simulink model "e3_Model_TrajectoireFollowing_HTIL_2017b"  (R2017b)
settings: Solver=FixedStepAuto  StartTime=0.0  StopTime=100  FixedStep=sampleTime  RelTol=1e-3  EnableMultiTasking=on
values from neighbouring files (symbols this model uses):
  k_d_x = 1.5    [StartSimulation.m]    (also in startSimulation.m; start.m = 1.65)
  k_d_y = 1.5    [StartSimulation.m]    (also in startSimulation.m; start.m = 1.52)
  k_d_yaw = 1    [StartSimulation.m]    (also in startSimulation.m; start.m)
  k_d_z = 0.5    [StartSimulation.m]    (also in startSimulation.m; start.m)
  k_i_x = 0.01    [StartSimulation.m]    (also in startSimulation.m; start.m = 0.9)
  k_i_y = 0.01    [StartSimulation.m]    (also in startSimulation.m; start.m = 0.91)
  k_i_yaw = 0.01    [StartSimulation.m]    (also in startSimulation.m; start.m)
  k_i_z = 0.01    [StartSimulation.m]    (also in startSimulation.m; start.m)
  k_p_x = 1.2    [StartSimulation.m]    (also in startSimulation.m; start.m = 1.9)
  k_p_y = 1.5    [StartSimulation.m]    (also in startSimulation.m; start.m = 1.9)
  k_p_yaw = 2    [StartSimulation.m]    (also in startSimulation.m; start.m)
  k_p_z = 2    [StartSimulation.m]    (also in startSimulation.m; start.m)
  saturation_psi = 2    [StartSimulation.m]    (also in startSimulation.m; start.m)
  saturation_x = 2    [StartSimulation.m]    (also in startSimulation.m; start.m)
  saturation_y = 2    [StartSimulation.m]    (also in startSimulation.m; start.m)
  saturation_z = 2    [StartSimulation.m]    (also in startSimulation.m; start.m)
libraries: simulink x37, aerolibanimutils x2, etargetslib x2

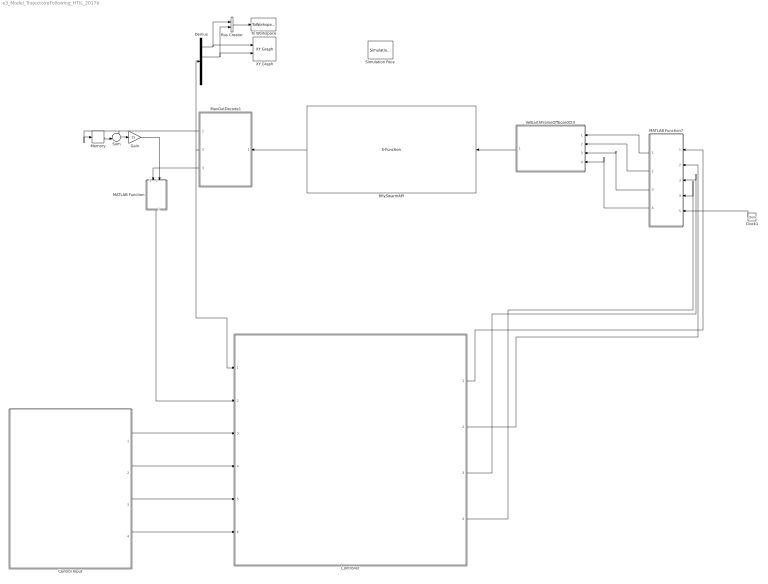
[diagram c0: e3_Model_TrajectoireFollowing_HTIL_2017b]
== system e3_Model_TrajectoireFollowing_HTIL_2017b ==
  Bus Creator : BusCreator  Inputs=2
  Clock1 : Clock
  Control Input : Subsystem
  Controller : Subsystem
  Demux : Demux
  Gain : Gain  Gain=25
  MATLAB Function : MATLAB Function  TreatAsAtomicUnit=on
  MATLAB Function7 : MATLAB Function  TreatAsAtomicUnit=on
  MavOutDecode1 : MATLAB Function  TreatAsAtomicUnit=on
  Memory : Memory
  RflySwarmAPI : S-Function  FunctionName=RflyUdpFast  Parameters=port,num,modeValue,T,ip  SFunctionDeploymentMode=off  EnableBusSupport=off  mask(UDP Receive){ip=255.255.255.255, port=20100, num=1, mode=FullData Mode, T=1/25, modeValue=0}
      mask prompts: ip "UDP IP Address"; port "UDP Port"; num "vehicle Number"; mode "UDP Mode"; T "Sample Time"
      mask help: This block receives bytes from an UDP/IP connection. The first parameter is the UDP port on the first CopterSim App The second parameter is the total vehicle number The third parameter is the data mode. check the help button for the definition
      mask init:
      | if strcmp(mode,'FullData Mode')
      |     modeValue = 0;
      | elseif strcmp(mode,'SimpleData Mode') 
      |     modeValue = 1;
      | elseif strcmp(mode,'UltraSimple Mode') 
      |     modeValue = 2;
      | else
      |     modeValue = 0;
      | end
  Simulation Pace : aerolibanimutils/Simulation Pace  SimulationPace=1  SleepMode=MATLAB Thread  OutputPaceError=off  SampleTime=-1
  Sum : Sum  Inputs=+-|
  To Workspace : ToWorkspace  VariableName=Pos  SaveFormat=Timeseries  SampleTime=-1
  VelEarthFrameOffboardCtrl : Subsystem
  XY Graph : simulink/Sinks/XY Graph  xmin=-1  xmax=1  ymin=-1  ymax=1  st=-1
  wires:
  Controller/1(Controller Output X) -> MATLAB Function7/1(X)
  Controller/2(Controller Output Y) -> MATLAB Function7/2(Y)
  Controller/3(Controller Output H) -> MATLAB Function7/3(H)
  Controller/4(Controller Output Psi) -> MATLAB Function7/4(Psi)
  Control Input/1(ux) -> Controller/3(Control input X)
  Control Input/2(uy) -> Controller/4(Control input Y)
  Control Input/3(uz) -> Controller/5(Control input H)
  Control Input/4(upsi) -> Controller/6(Control input Psi)
  RflySwarmAPI/1 -> MavOutDecode1/1(u)
  VelEarthFrameOffboardCtrl/1(Out1) -> RflySwarmAPI/1
  Clock1/1 -> MATLAB Function7/5(t)
  MATLAB Function7/4(p1) -> VelEarthFrameOffboardCtrl/4(yawRate_rads)
  MATLAB Function7/3(h1) -> VelEarthFrameOffboardCtrl/3(VeZ_ms)
  MATLAB Function7/2(y1) -> VelEarthFrameOffboardCtrl/2(VeY_ms)
  MATLAB Function7/1(x1) -> VelEarthFrameOffboardCtrl/1(VeX_ms)
  MavOutDecode1/2(localPos) -> Demux/1, Controller/1(Feedback Position)
  Demux/1 -> Bus Creator/1, XY Graph/1
  Demux/2 -> Bus Creator/2, XY Graph/2
  MavOutDecode1/1(Psi) -> Memory/1, Sum/1
  Memory/1 -> Sum/2
  Sum/1 -> Gain/1
  Gain/1 -> MATLAB Function/2(psi)
  MavOutDecode1/3(localVel) -> MATLAB Function/1(v)
  MATLAB Function/1(y) -> Controller/2(Feedback Velocity)
  Bus Creator/1 -> To Workspace/1

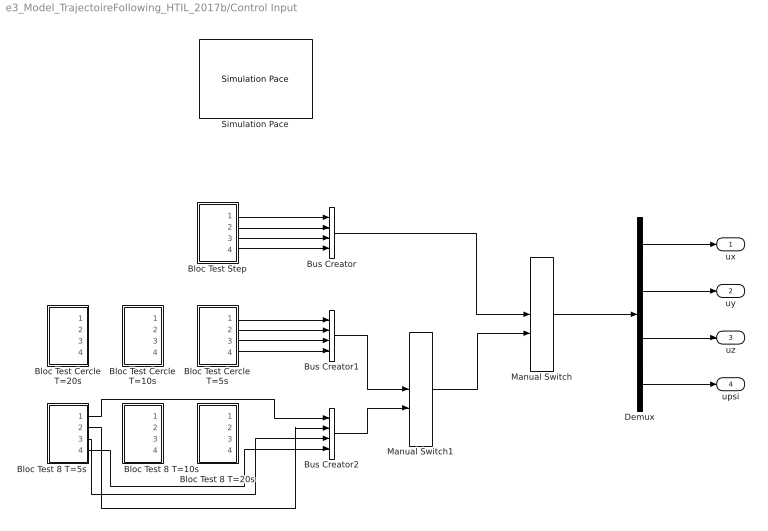
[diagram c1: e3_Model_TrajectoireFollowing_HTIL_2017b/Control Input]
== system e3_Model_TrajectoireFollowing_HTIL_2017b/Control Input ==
  Bloc Test 8 T=10s : Subsystem
  Bloc Test 8 T=20s : Subsystem
  Bloc Test 8 T=5s : Subsystem
  Bloc Test Cercle T=10s : Subsystem
  Bloc Test Cercle T=20s : Subsystem
  Bloc Test Cercle T=5s : Subsystem
  Bloc Test Step : Subsystem
  Bus Creator : BusCreator  Inputs=4
  Bus Creator1 : BusCreator  Inputs=4
  Bus Creator2 : BusCreator  Inputs=4
  Demux : Demux
  Manual Switch : ManualSwitch  CurrentSetting=0
  Manual Switch1 : ManualSwitch
  Simulation Pace : aerolibanimutils/Simulation Pace  Commented=on  SimulationPace=100  SleepMode=MATLAB Thread  OutputPaceError=off  SampleTime=-1
  ux : Outport
  uy : Outport  Port=2
  uz : Outport  Port=3
  upsi : Outport  Port=4
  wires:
  Demux/2 -> uy/1
  Demux/1 -> ux/1
  Bloc Test Step/2(uy) -> Bus Creator/2
  Demux/3 -> uz/1
  Demux/4 -> upsi/1
  Bloc Test Step/4(upsi) -> Bus Creator/4
  Bloc Test Step/3(uz) -> Bus Creator/3
  Bloc Test Step/1(ux) -> Bus Creator/1
  Bus Creator/1 -> Manual Switch/1
  Bus Creator1/1 -> Manual Switch1/1
  Bus Creator2/1 -> Manual Switch1/2
  Manual Switch/1 -> Demux/1
  Manual Switch1/1 -> Manual Switch/2
  Bloc Test 8 T=5s/1(ux) -> Bus Creator2/1
  Bloc Test 8 T=5s/2(uy) -> Bus Creator2/2
  Bloc Test 8 T=5s/3(uz) -> Bus Creator2/3
  Bloc Test 8 T=5s/4(upsi) -> Bus Creator2/4
  Bloc Test Cercle T=5s/1(ux) -> Bus Creator1/1
  Bloc Test Cercle T=5s/2(uy) -> Bus Creator1/2
  Bloc Test Cercle T=5s/3(uz) -> Bus Creator1/3
  Bloc Test Cercle T=5s/4(upsi) -> Bus Creator1/4

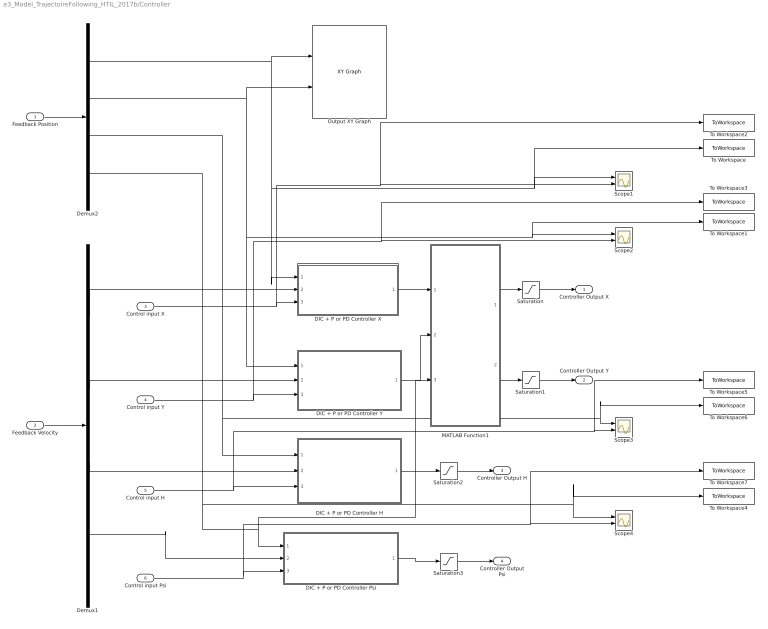
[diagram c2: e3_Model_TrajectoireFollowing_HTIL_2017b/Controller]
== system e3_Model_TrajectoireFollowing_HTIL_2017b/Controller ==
  Feedback Position : Inport
  Feedback Velocity : Inport  Port=2
  Control input X : Inport  Port=3
  Control input Y : Inport  Port=4
  Control input H : Inport  Port=5
  Control input Psi : Inport  Port=6
  DIC + P or PD Controller H : Subsystem
  DIC + P or PD Controller Psi : Subsystem
  DIC + P or PD Controller X : Subsystem
  DIC + P or PD Controller Y : Subsystem
  Demux1 : Demux
  Demux2 : Demux
  MATLAB Function1 : MATLAB Function  TreatAsAtomicUnit=on
  Output XY Graph : simulink/Sinks/XY Graph  Commented=on  xmin=-5  xmax=5  ymin=-5  ymax=5  st=-1
  Saturation : Saturate  UpperLimit=saturation_x  LowerLimit=-saturation_x
  Saturation1 : Saturate  UpperLimit=saturation_y  LowerLimit=-saturation_y
  Saturation2 : Saturate  UpperLimit=saturation_z  LowerLimit=-saturation_z
  Saturation3 : Saturate  UpperLimit=saturation_psi  LowerLimit=-saturation_psi
  Scope{1..4} (4 alike) : Scope  NumInputPorts=2
  To Workspace : ToWorkspace  VariableName=N4_Step1_Out_X  SampleTime=-1
  To Workspace1 : ToWorkspace  VariableName=N4_Step1_Out_Y  SampleTime=-1
  To Workspace2 : ToWorkspace  VariableName=N4_Step1_In_X  SampleTime=-1
  To Workspace3 : ToWorkspace  VariableName=N4_Step1_In_Y  SampleTime=-1
  To Workspace4 : ToWorkspace  VariableName=N4_Step1_Out_Psi  SampleTime=-1
  To Workspace5 : ToWorkspace  VariableName=N4_Step1_In_H  SampleTime=-1
  To Workspace6 : ToWorkspace  VariableName=N4_Step1_Out_H  SampleTime=-1
  To Workspace7 : ToWorkspace  VariableName=N4_Step1_In_Psi  SampleTime=-1
  Controller Output X : Outport
  Controller Output Y : Outport  Port=2
  Controller Output H : Outport  Port=3
  Controller Output Psi : Outport  Port=4
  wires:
  Feedback Position/1 -> Demux2/1
  Feedback Velocity/1 -> Demux1/1
  Demux1/2 -> DIC + P or PD Controller Y/2(Feedback Velocity Y)
  Demux2/3 -> Scope3/1, To Workspace6/1, DIC + P or PD Controller H/1(Feedback Position H)
  Demux1/1 -> DIC + P or PD Controller X/2(Feedback Velocity X)
  Demux1/3 -> DIC + P or PD Controller H/2(Feedback Velocity H)
  Control input X/1 -> To Workspace2/1, Scope1/2, DIC + P or PD Controller X/3(Control Input X)
  Control input H/1 -> Scope3/2, To Workspace5/1, DIC + P or PD Controller H/3(Control Input H)
  Saturation/1 -> Controller Output X/1
  Saturation1/1 -> Controller Output Y/1
  Saturation2/1 -> Controller Output H/1
  Saturation3/1 -> Controller Output Psi/1
  Control input Y/1 -> Scope2/2, To Workspace3/1, DIC + P or PD Controller Y/3(Control Input Y)
  DIC + P or PD Controller H/1(Controller Output H) -> Saturation2/1
  DIC + P or PD Controller Psi/1(Controller Output Psi) -> Saturation3/1
  Demux2/1 -> DIC + P or PD Controller X/1(Feedback Position X), To Workspace/1, Scope1/1, Output XY Graph/1
  Demux2/2 -> Scope2/1, To Workspace1/1, DIC + P or PD Controller Y/1(Feedback Position Y), Output XY Graph/2
  Demux2/4 -> Scope4/1, To Workspace4/1, MATLAB Function1/3(psi), DIC + P or PD Controller Psi/1(Feedback Position Psi)
  Demux1/4 -> DIC + P or PD Controller Psi/2(Feedback Velocity Psi)
  Control input Psi/1 -> Scope4/2, To Workspace7/1, DIC + P or PD Controller Psi/3(Control input Psi)
  DIC + P or PD Controller Y/1(Controller Output Y) -> MATLAB Function1/2(eay)
  MATLAB Function1/2(y) -> Saturation1/1
  DIC + P or PD Controller X/1(Controller Output X) -> MATLAB Function1/1(eax)
  MATLAB Function1/1(x) -> Saturation/1

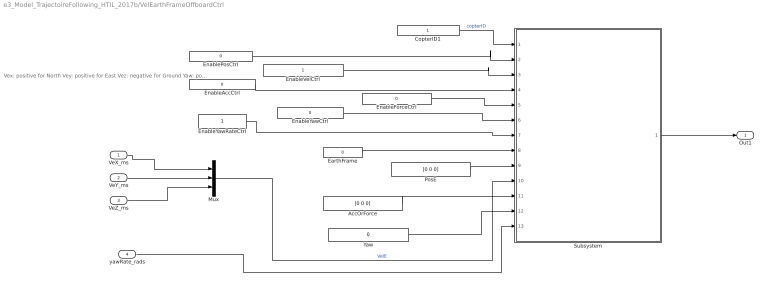
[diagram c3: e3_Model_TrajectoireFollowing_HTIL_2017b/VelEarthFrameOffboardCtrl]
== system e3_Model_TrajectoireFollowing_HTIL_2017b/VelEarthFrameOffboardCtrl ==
  note: Vex: positive for North Vey: positive for East Vez: negative for Ground Yaw: positive for right rotation
  VeX_ms : Inport
  VeY_ms : Inport  Port=2
  VeZ_ms : Inport  Port=3
  yawRate_rads : Inport  Port=4  PortDimensions=1
  AccOrForce : Constant  Value=[0 0 0]
  CopterID1 : Constant
  EarthFrame : Constant  Value=0
  EnableAccCtrl : Constant  Value=0
  EnableForceCtrl : Constant  Value=0
  EnablePosCtrl : Constant  Value=0
  EnableVelCtrl : Constant
  EnableYawCtrl : Constant  Value=0
  EnableYawRateCtrl : Constant
  Mux : Mux  Inputs=3
  PosE : Constant  Value=[0 0 0]
  Subsystem : Subsystem
  Yaw : Constant  Value=0
  Out1 : Outport  VectorParamsAs1DForOutWhenUnconnected=on
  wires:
  Yaw/1 -> Subsystem/12(yaw)
  EnableYawRateCtrl/1 -> Subsystem/7(EnYawrate)
  EnableYawCtrl/1 -> Subsystem/6(enYaw)
  EnableAccCtrl/1 -> Subsystem/4(enAcc)
  Mux/1 -> Subsystem/10(vel)  "VelE"
  EarthFrame/1 -> Subsystem/8(FrameIndex)
  yawRate_rads/1 -> Subsystem/13(yawrate)
  AccOrForce/1 -> Subsystem/11(acc)
  EnableVelCtrl/1 -> Subsystem/3(enVel)
  EnableForceCtrl/1 -> Subsystem/5(enForce)
  CopterID1/1 -> Subsystem/1(CopterID)  "copterID"
  EnablePosCtrl/1 -> Subsystem/2(enPos)
  PosE/1 -> Subsystem/9(pos)
  VeY_ms/1 -> Mux/2
  VeX_ms/1 -> Mux/1
  VeZ_ms/1 -> Mux/3
  Subsystem/1(Out1) -> Out1/1

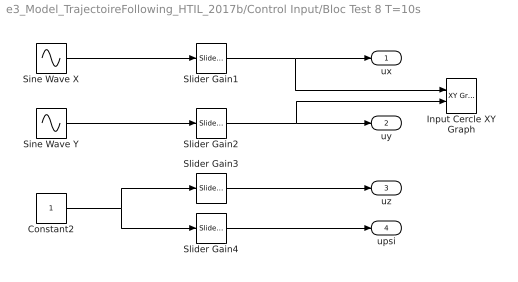
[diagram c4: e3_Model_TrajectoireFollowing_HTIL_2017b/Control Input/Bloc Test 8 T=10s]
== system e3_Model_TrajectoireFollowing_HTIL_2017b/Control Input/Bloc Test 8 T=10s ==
  Constant2 : Constant
  Input Cercle XY Graph : simulink/Sinks/XY Graph  Commented=on  xmin=-2  xmax=2  ymin=-2  ymax=2  st=-1
  Sine Wave X : Sin  Frequency=0.104  SampleTime=0
  Sine Wave Y : Sin  Frequency=0.104  SampleTime=0
  Slider Gain1 : simulink/Math Operations/Slider Gain  gain=1  low=-10  high=10
  Slider Gain2 : simulink/Math Operations/Slider Gain  gain=1  low=-10  high=10
  Slider Gain3 : simulink/Math Operations/Slider Gain  gain=1  low=-3  high=3
  Slider Gain4 : simulink/Math Operations/Slider Gain  gain=0  low=-2  high=2
  ux : Outport
  uy : Outport  Port=2
  uz : Outport  Port=3
  upsi : Outport  Port=4
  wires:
  Slider Gain2/1 -> Input Cercle XY Graph/2, uy/1
  Slider Gain3/1 -> uz/1
  Slider Gain4/1 -> upsi/1
  Slider Gain1/1 -> Input Cercle XY Graph/1, ux/1
  Constant2/1 -> Slider Gain4/1, Slider Gain3/1
  Sine Wave Y/1 -> Slider Gain2/1
  Sine Wave X/1 -> Slider Gain1/1

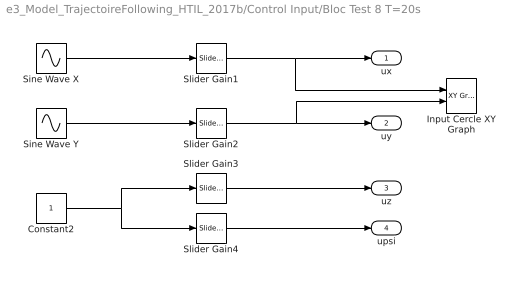
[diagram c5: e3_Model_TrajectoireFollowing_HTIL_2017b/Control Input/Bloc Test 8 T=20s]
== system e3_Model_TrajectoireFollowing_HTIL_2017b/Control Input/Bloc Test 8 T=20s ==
  Constant2 : Constant
  Input Cercle XY Graph : simulink/Sinks/XY Graph  Commented=on  xmin=-2  xmax=2  ymin=-2  ymax=2  st=-1
  Sine Wave X : Sin  Frequency=0.104  SampleTime=0
  Sine Wave Y : Sin  Frequency=0.104  SampleTime=0
  Slider Gain1 : simulink/Math Operations/Slider Gain  gain=1  low=-10  high=10
  Slider Gain2 : simulink/Math Operations/Slider Gain  gain=1  low=-10  high=10
  Slider Gain3 : simulink/Math Operations/Slider Gain  gain=1  low=-3  high=3
  Slider Gain4 : simulink/Math Operations/Slider Gain  gain=0  low=-2  high=2
  ux : Outport
  uy : Outport  Port=2
  uz : Outport  Port=3
  upsi : Outport  Port=4
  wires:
  Slider Gain2/1 -> Input Cercle XY Graph/2, uy/1
  Slider Gain3/1 -> uz/1
  Slider Gain4/1 -> upsi/1
  Slider Gain1/1 -> Input Cercle XY Graph/1, ux/1
  Constant2/1 -> Slider Gain4/1, Slider Gain3/1
  Sine Wave Y/1 -> Slider Gain2/1
  Sine Wave X/1 -> Slider Gain1/1

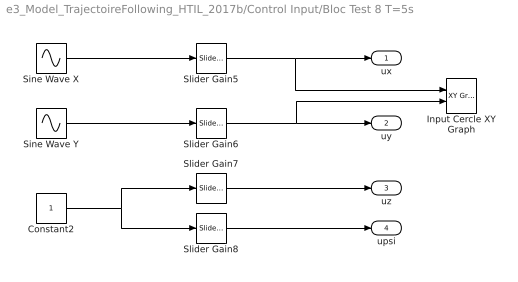
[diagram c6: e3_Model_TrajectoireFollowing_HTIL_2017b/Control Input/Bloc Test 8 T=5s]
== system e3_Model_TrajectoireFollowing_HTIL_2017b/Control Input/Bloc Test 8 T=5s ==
  Constant2 : Constant
  Input Cercle XY Graph : simulink/Sinks/XY Graph  Commented=on  xmin=-2  xmax=2  ymin=-2  ymax=2  st=-1
  Sine Wave X : Sin  SampleTime=0
  Sine Wave Y : Sin  Frequency=2  SampleTime=0
  Slider Gain5 : simulink/Math Operations/Slider Gain  gain=1  low=-10  high=10
  Slider Gain6 : simulink/Math Operations/Slider Gain  gain=1  low=-10  high=10
  Slider Gain7 : simulink/Math Operations/Slider Gain  gain=1  low=-3  high=3
  Slider Gain8 : simulink/Math Operations/Slider Gain  gain=0  low=-2  high=2
  ux : Outport
  uy : Outport  Port=2
  uz : Outport  Port=3
  upsi : Outport  Port=4
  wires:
  Slider Gain6/1 -> Input Cercle XY Graph/2, uy/1
  Slider Gain7/1 -> uz/1
  Slider Gain8/1 -> upsi/1
  Slider Gain5/1 -> Input Cercle XY Graph/1, ux/1
  Constant2/1 -> Slider Gain8/1, Slider Gain7/1
  Sine Wave Y/1 -> Slider Gain6/1
  Sine Wave X/1 -> Slider Gain5/1

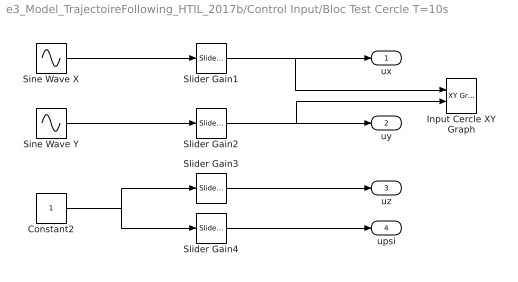
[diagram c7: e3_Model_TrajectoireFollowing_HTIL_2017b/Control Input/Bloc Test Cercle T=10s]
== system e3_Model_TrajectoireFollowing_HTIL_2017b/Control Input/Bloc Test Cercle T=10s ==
  Constant2 : Constant
  Input Cercle XY Graph : simulink/Sinks/XY Graph  Commented=on  xmin=-2  xmax=2  ymin=-2  ymax=2  st=-1
  Sine Wave X : Sin  Frequency=0.65  SampleTime=0
  Sine Wave Y : Sin  Frequency=0.65  Phase=pi/2  SampleTime=0
  Slider Gain1 : simulink/Math Operations/Slider Gain  gain=2.0  low=-10  high=10
  Slider Gain2 : simulink/Math Operations/Slider Gain  gain=2  low=-10  high=10
  Slider Gain3 : simulink/Math Operations/Slider Gain  gain=1  low=-3  high=3
  Slider Gain4 : simulink/Math Operations/Slider Gain  gain=0  low=-2  high=2
  ux : Outport
  uy : Outport  Port=2
  uz : Outport  Port=3
  upsi : Outport  Port=4
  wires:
  Slider Gain2/1 -> Input Cercle XY Graph/2, uy/1
  Slider Gain3/1 -> uz/1
  Slider Gain4/1 -> upsi/1
  Slider Gain1/1 -> Input Cercle XY Graph/1, ux/1
  Constant2/1 -> Slider Gain4/1, Slider Gain3/1
  Sine Wave Y/1 -> Slider Gain2/1
  Sine Wave X/1 -> Slider Gain1/1

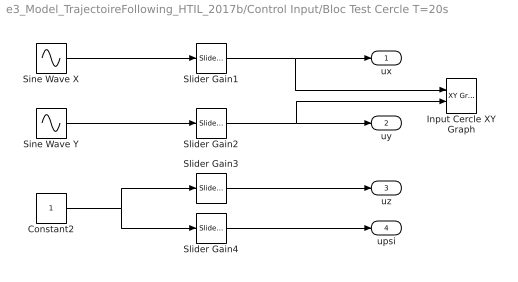
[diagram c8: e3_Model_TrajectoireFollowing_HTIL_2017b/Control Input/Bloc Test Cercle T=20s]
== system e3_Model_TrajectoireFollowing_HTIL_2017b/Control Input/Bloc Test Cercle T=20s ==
  Constant2 : Constant
  Input Cercle XY Graph : simulink/Sinks/XY Graph  Commented=on  xmin=-2  xmax=2  ymin=-2  ymax=2  st=-1
  Sine Wave X : Sin  Frequency=0.35  SampleTime=0
  Sine Wave Y : Sin  Frequency=0.35  Phase=pi/2  SampleTime=0
  Slider Gain1 : simulink/Math Operations/Slider Gain  gain=2  low=-10  high=10
  Slider Gain2 : simulink/Math Operations/Slider Gain  gain=2  low=-10  high=10
  Slider Gain3 : simulink/Math Operations/Slider Gain  gain=1  low=-3  high=3
  Slider Gain4 : simulink/Math Operations/Slider Gain  gain=0  low=-2  high=2
  ux : Outport
  uy : Outport  Port=2
  uz : Outport  Port=3
  upsi : Outport  Port=4
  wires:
  Slider Gain2/1 -> Input Cercle XY Graph/2, uy/1
  Slider Gain3/1 -> uz/1
  Slider Gain4/1 -> upsi/1
  Slider Gain1/1 -> Input Cercle XY Graph/1, ux/1
  Constant2/1 -> Slider Gain4/1, Slider Gain3/1
  Sine Wave Y/1 -> Slider Gain2/1
  Sine Wave X/1 -> Slider Gain1/1

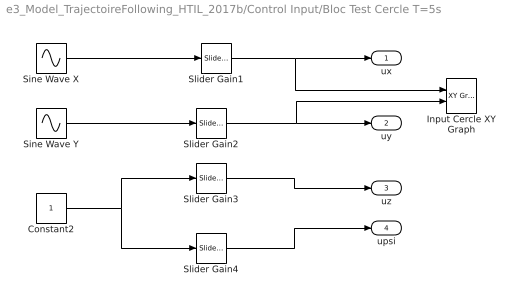
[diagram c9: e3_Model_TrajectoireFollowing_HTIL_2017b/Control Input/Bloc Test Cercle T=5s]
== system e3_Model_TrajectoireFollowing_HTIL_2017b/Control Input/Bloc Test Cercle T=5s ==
  Constant2 : Constant
  Input Cercle XY Graph : simulink/Sinks/XY Graph  Commented=on  xmin=-2  xmax=2  ymin=-2  ymax=2  st=-1
  Sine Wave X : Sin  SampleTime=0
  Sine Wave Y : Sin  Phase=pi/2  SampleTime=0
  Slider Gain1 : simulink/Math Operations/Slider Gain  gain=2  low=-10  high=10
  Slider Gain2 : simulink/Math Operations/Slider Gain  gain=2  low=-10  high=10
  Slider Gain3 : simulink/Math Operations/Slider Gain  gain=1  low=-3  high=3
  Slider Gain4 : simulink/Math Operations/Slider Gain  gain=0  low=-2  high=2
  ux : Outport
  uy : Outport  Port=2
  uz : Outport  Port=3
  upsi : Outport  Port=4
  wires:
  Slider Gain2/1 -> Input Cercle XY Graph/2, uy/1
  Slider Gain3/1 -> uz/1
  Slider Gain4/1 -> upsi/1
  Slider Gain1/1 -> Input Cercle XY Graph/1, ux/1
  Constant2/1 -> Slider Gain4/1, Slider Gain3/1
  Sine Wave Y/1 -> Slider Gain2/1
  Sine Wave X/1 -> Slider Gain1/1

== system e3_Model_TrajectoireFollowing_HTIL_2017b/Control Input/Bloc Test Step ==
  Constant2 : Constant
  Input Segment XY Graph : simulink/Sinks/XY Graph  Commented=on  xmin=-2  xmax=2  ymin=-2  ymax=2  st=-1
  Slider Gain1 : simulink/Math Operations/Slider Gain  gain=1  low=-10  high=10
  Slider Gain2 : simulink/Math Operations/Slider Gain  gain=1  low=-10  high=10
  Slider Gain3 : simulink/Math Operations/Slider Gain  gain=1  low=-2  high=2
  Slider Gain4 : simulink/Math Operations/Slider Gain  gain=0  low=-2  high=2
  Step X1 : Step  Time=5  SampleTime=0
  ux : Outport
  uy : Outport  Port=2
  uz : Outport  Port=3
  upsi : Outport  Port=4
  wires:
  Slider Gain1/1 -> Input Segment XY Graph/1, ux/1
  Slider Gain2/1 -> Input Segment XY Graph/2, uy/1
  Slider Gain3/1 -> uz/1
  Slider Gain4/1 -> upsi/1
  Step X1/1 -> Slider Gain3/1, Slider Gain4/1, Slider Gain2/1, Slider Gain1/1

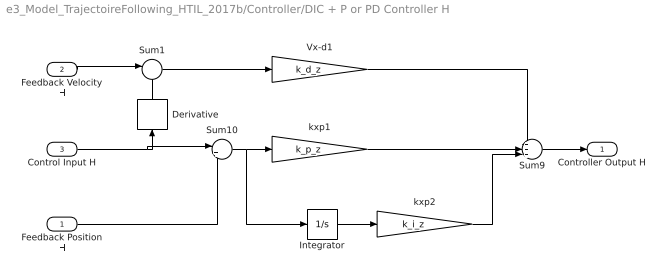
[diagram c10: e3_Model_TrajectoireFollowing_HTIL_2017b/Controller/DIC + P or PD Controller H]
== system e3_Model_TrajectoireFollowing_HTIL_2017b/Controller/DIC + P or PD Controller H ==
  Feedback Position H : Inport
  Feedback Velocity H : Inport  Port=2
  Control Input H : Inport  Port=3
  Derivative : Derivative
  Integrator : Integrator
  Sum1 : Sum  Inputs=|-+
  Sum10 : Sum  Inputs=|+-
  Sum9 : Sum  Inputs=+++|
  Vx-d1 : Gain  Gain=k_d_z
  kxp1 : Gain  Gain=k_p_z
  kxp2 : Gain  Gain=k_i_z
  Controller Output H : Outport
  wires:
  Sum9/1 -> Controller Output H/1
  Sum10/1 -> Integrator/1, kxp1/1
  kxp1/1 -> Sum9/2
  Vx-d1/1 -> Sum9/1
  Feedback Velocity H/1 -> Sum1/1
  Sum1/1 -> Vx-d1/1
  Integrator/1 -> kxp2/1
  kxp2/1 -> Sum9/3
  Control Input H/1 -> Sum10/1, Derivative/1
  Feedback Position H/1 -> Sum10/2
  Derivative/1 -> Sum1/2

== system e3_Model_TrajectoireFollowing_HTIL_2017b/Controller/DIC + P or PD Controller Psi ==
  Feedback Position Psi : Inport
  Feedback Velocity Psi : Inport  Port=2
  Control input Psi : Inport  Port=3
  Derivative : Derivative
  Gain : Gain  Gain=k_p_yaw
  Gain1 : Gain  Gain=k_d_yaw
  Integrator : Integrator
  Sum1 : Sum  Inputs=|-+
  Sum10 : Sum  Inputs=|+-
  Sum9 : Sum  Inputs=+++|
  kxp2 : Gain  Gain=k_i_yaw
  Controller Output Psi : Outport
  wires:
  Sum9/1 -> Controller Output Psi/1
  kxp2/1 -> Sum9/3
  Control input Psi/1 -> Sum10/1, Derivative/1
  Gain1/1 -> Sum9/1
  Sum10/1 -> Gain/1, Integrator/1
  Integrator/1 -> kxp2/1
  Feedback Velocity Psi/1 -> Sum1/1
  Sum1/1 -> Gain1/1
  Gain/1 -> Sum9/2
  Derivative/1 -> Sum1/2
  Feedback Position Psi/1 -> Sum10/2

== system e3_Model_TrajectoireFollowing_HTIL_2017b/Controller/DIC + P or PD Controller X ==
  Feedback Position X : Inport
  Feedback Velocity X : Inport  Port=2
  Control Input X : Inport  Port=3
  Derivative : Derivative
  Integrator : Integrator
  Sum1 : Sum  Inputs=|-+
  Sum10 : Sum  Inputs=|+-
  Sum9 : Sum  Inputs=+++|
  Vx-d3 : Gain  Gain=k_d_x
  kxp2 : Gain  Gain=k_i_x
  kxp3 : Gain  Gain=k_p_x
  Controller Output X : Outport
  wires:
  Sum9/1 -> Controller Output X/1
  Feedback Velocity X/1 -> Sum1/1
  Feedback Position X/1 -> Sum10/2
  Sum1/1 -> Vx-d3/1
  Integrator/1 -> kxp2/1
  kxp3/1 -> Sum9/2
  Vx-d3/1 -> Sum9/1
  Sum10/1 -> kxp3/1, Integrator/1
  Derivative/1 -> Sum1/2
  kxp2/1 -> Sum9/3
  Control Input X/1 -> Sum10/1, Derivative/1

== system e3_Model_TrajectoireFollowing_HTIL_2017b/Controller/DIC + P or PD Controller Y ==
  Feedback Position Y : Inport
  Feedback Velocity Y : Inport  Port=2
  Control Input Y : Inport  Port=3
  Derivative : Derivative
  Integrator : Integrator
  Sum1 : Sum  Inputs=|-+
  Sum10 : Sum  Inputs=|+-
  Sum9 : Sum  Inputs=+++|
  Vx-d3 : Gain  Gain=k_d_y
  kxp2 : Gain  Gain=k_i_y
  kxp3 : Gain  Gain=k_p_y
  Controller Output Y : Outport
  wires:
  Feedback Position Y/1 -> Sum10/2
  Control Input Y/1 -> Sum10/1, Derivative/1
  Sum9/1 -> Controller Output Y/1
  Integrator/1 -> kxp2/1
  kxp3/1 -> Sum9/2
  Sum10/1 -> kxp3/1, Integrator/1
  kxp2/1 -> Sum9/3
  Vx-d3/1 -> Sum9/1
  Feedback Velocity Y/1 -> Sum1/1
  Sum1/1 -> Vx-d3/1
  Derivative/1 -> Sum1/2

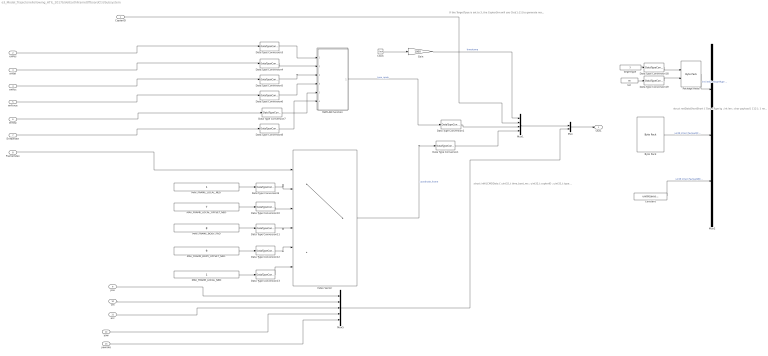
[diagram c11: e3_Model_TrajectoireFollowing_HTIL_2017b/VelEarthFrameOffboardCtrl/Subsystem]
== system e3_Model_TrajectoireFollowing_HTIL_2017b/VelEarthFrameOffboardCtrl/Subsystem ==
  note: struct netDataShortShort { TargetType tg ; int len ; char payload [ 112 ]; } netDataShortShort ;
  note: struct inHILCMDData { uint32_t time_boot_ms ; uint32_t copterID ; uint32_t type_mask ; uint32_t coordinate_frame ; float ctrls [ 11 ]; };
  note: If the TargetTpye is set to 3, the CopterSim will use Ctrs[1:11] to generate mavlink S ET_POSITION_TARGET_LOCAL_NED msg to UAV's Offboard mode Control， If the PX4 is not armed, CopterSim will send the arm command repeatly. If the PX4 is not in Offboard(Guided) Mode, CopterSim will send SET_MODE msg repeatly.
  CopterID : Inport
  enPos : Inport  Port=2
  enVel : Inport  Port=3
  enAcc : Inport  Port=4
  enForce : Inport  Port=5
  enYaw : Inport  Port=6
  EnYawrate : Inport  Port=7
  FrameIndex : Inport  Port=8
  pos : Inport  Port=9  PortDimensions=3
  vel : Inport  Port=10  PortDimensions=3
  acc : Inport  Port=11  PortDimensions=3
  yaw : Inport  Port=12  PortDimensions=1
  yawrate : Inport  Port=13  PortDimensions=1
  Byte Pack : etargetslib/Byte Pack  Commented=on  datatypes={'uint32','single'}  byteAlign=1
  Clock : Clock
  Constant : Constant  Commented=on  Value=uint8(zeros(32,1))
  Data Type Conversion : DataTypeConversion  OutDataTypeStr=double
  Data Type Conversion1 : DataTypeConversion  OutDataTypeStr=double
  Data Type Conversion{9..13} (5 alike) : DataTypeConversion  OutDataTypeStr=uint8
  Data Type Conversion18 : DataTypeConversion  Commented=on  OutDataTypeStr=uint32
  Data Type Conversion19 : DataTypeConversion  Commented=on  OutDataTypeStr=int32
  Data Type Conversion{3..8} (6 alike) : DataTypeConversion  OutDataTypeStr=boolean
  Gain : Gain  Gain=1000
  Index Vector : MultiPortSwitch  DataPortOrder=Zero-based contiguous  Inputs=5  zeroidx=on
  MATLAB Function : MATLAB Function  TreatAsAtomicUnit=on
  MAV_FRAME_BODY_FRD : Constant  Value=8
  "MAV_FRAME_BODY_OFFSET_NED " : Constant  Value=9
  MAV_FRAME_LOCAL_NED : Constant
  "MAV_FRAME_LOCAL_NED " : Constant
  MAV_FRAME_LOCAL_OFFSET_NED : Constant  Value=7
  Mux : Mux  Inputs=2
  Mux1 : Mux
  Mux2 : Mux  Commented=on  Inputs=3
  Mux5 : Mux  Inputs=5
  Package Head : etargetslib/Byte Pack  Commented=on  datatypes={'uint32','int32'}  byteAlign=4
  TargetType : Constant  Commented=on  Value=3  OutDataTypeStr=Inherit: Inherit via back propagation
  len : Constant  Commented=on  Value=80  OutDataTypeStr=Inherit: Inherit via back propagation
  Out1 : Outport  VectorParamsAs1DForOutWhenUnconnected=on
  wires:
  Data Type Conversion7/1 -> MATLAB Function/5(Yaw)
  Data Type Conversion6/1 -> MATLAB Function/4(Force)
  vel/1 -> Mux5/2
  MAV_FRAME_BODY_FRD/1 -> Data Type Conversion11/1
  Data Type Conversion3/1 -> MATLAB Function/1(pos)
  Data Type Conversion5/1 -> MATLAB Function/3(Acc)
  Data Type Conversion4/1 -> MATLAB Function/2(vel)
  Data Type Conversion8/1 -> MATLAB Function/6(Yawrate)
  enAcc/1 -> Data Type Conversion5/1
  enYaw/1 -> Data Type Conversion7/1
  EnYawrate/1 -> Data Type Conversion8/1
  enForce/1 -> Data Type Conversion6/1
  "MAV_FRAME_LOCAL_NED "/1 -> Data Type Conversion9/1
  enPos/1 -> Data Type Conversion3/1
  Data Type Conversion9/1 -> Index Vector/2
  Data Type Conversion10/1 -> Index Vector/3
  Index Vector/1 -> Data Type Conversion/1  "coordinate_frame"
  Constant/1 -> Mux2/3  "uint8 (char) Payload[80:111]"
  Data Type Conversion18/1 -> Package Head/1
  Clock/1 -> Gain/1
  len/1 -> Data Type Conversion19/1
  Mux5/1 -> Mux/2
  MATLAB Function/1(y) -> Data Type Conversion1/1  "type_mask"
  Package Head/1 -> Mux2/1  "int (int32) TargetType & len"
  TargetType/1 -> Data Type Conversion18/1
  Gain/1 -> Mux1/1  "timestamp"
  Data Type Conversion19/1 -> Package Head/2
  pos/1 -> Mux5/1
  Byte Pack/1 -> Mux2/2  "uint8 (char) Payload[0:79]"
  Data Type Conversion13/1 -> Index Vector/6
  Data Type Conversion12/1 -> Index Vector/5
  acc/1 -> Mux5/3
  FrameIndex/1 -> Index Vector/1
  MAV_FRAME_LOCAL_NED/1 -> Data Type Conversion13/1
  MAV_FRAME_LOCAL_OFFSET_NED/1 -> Data Type Conversion10/1
  Data Type Conversion11/1 -> Index Vector/4
  "MAV_FRAME_BODY_OFFSET_NED "/1 -> Data Type Conversion12/1
  enVel/1 -> Data Type Conversion4/1
  yaw/1 -> Mux5/4
  yawrate/1 -> Mux5/5
  CopterID/1 -> Mux1/2
  Mux1/1 -> Mux/1
  Mux/1 -> Out1/1
  Data Type Conversion/1 -> Mux1/4
  Data Type Conversion1/1 -> Mux1/3

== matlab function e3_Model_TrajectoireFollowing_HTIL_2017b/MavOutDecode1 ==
function [Psi,localPos,localVel] = fcn(u)
localPos = [u(7:8);-u(9);u(6)];
localVel = u(10:12);
Psi=u(6);

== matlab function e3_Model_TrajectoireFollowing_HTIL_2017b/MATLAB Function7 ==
function [x1,y1,h1,p1] = fcn(X,Y,H,Psi,t)

% position1=[u(1,1);u(3,1);0];
% position2=[u(2,1);u(4,1);0];
if t<5
    x1=0;
    y1=0;
    h1=-1;
    p1=0;
else
    x1=X;
    y1=Y;
    h1=-H;
    p1=Psi;
   
end

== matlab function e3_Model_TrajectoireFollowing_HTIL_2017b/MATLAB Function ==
function y = fcn(v,psi)

y = [v;psi];

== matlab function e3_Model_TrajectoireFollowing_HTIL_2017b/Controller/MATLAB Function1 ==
function [x,y] = fcn(eax,eay,psi)
g=9.8;

theta =eax/g;% vx
phi =eay/g;% vy
R=[cos(psi),-sin(psi);
    sin(psi),cos(psi)];
u=R^(-1)*[theta;phi];
x=u(1);
y=u(2);

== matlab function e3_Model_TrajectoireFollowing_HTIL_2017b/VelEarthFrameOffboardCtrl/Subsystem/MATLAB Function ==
function y = fcn(pos,vel,Acc,Force,Yaw,Yawrate)
y=uint32(0);
if ~pos
    y = bitor(y,uint32(7));
end

if~vel
    y = bitor(y,bitshift(uint32(7),3));
end

if ~Acc
    y = bitor(y,bitshift(uint32(7),6));
end

if Force
    y = bitor(y,bitshift(uint32(1),9));
end

if ~Yaw
    y = bitor(y,bitshift(uint32(1),10));
end

if ~Yawrate
    y = bitor(y,bitshift(uint32(1),11));
end
